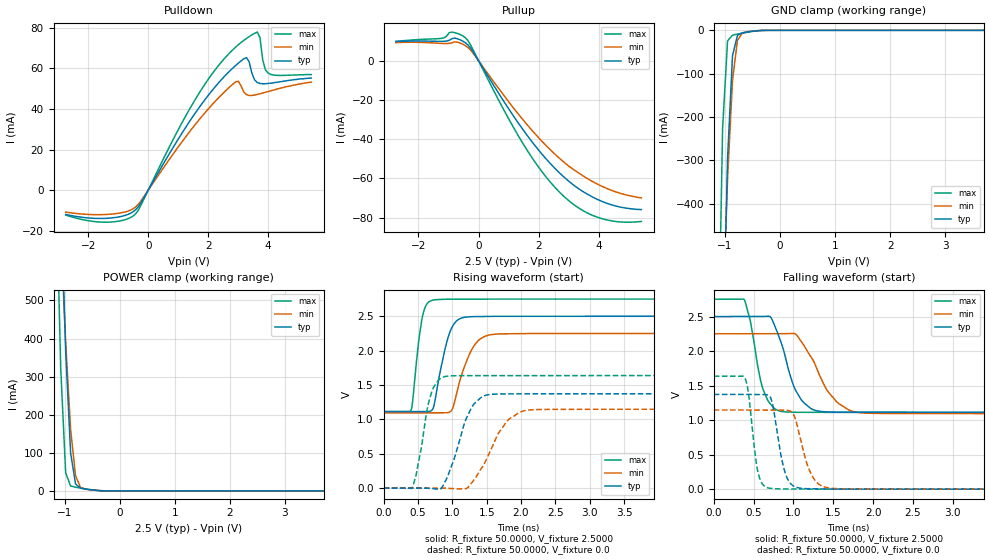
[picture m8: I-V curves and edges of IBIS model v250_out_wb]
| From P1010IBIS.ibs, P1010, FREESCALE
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[Model] v250_out_wb
|   Model v250_out_wb
| This model has derived from v250_wb
| Only applicable curves and parameters are copied
Model_type Output
Polarity   Non-Inverting
Enable   Active-High
Vmeas =  1.2500V
Cref =   0.0F
Rref =   50.0000
Vref =   1.2500V
C_comp   2.1221pF   1.9600pF   2.4667pF
[Temperature Range]   85.0000   0.1250k   -40.0000
[Voltage Range]   2.5000V   2.2500V   2.7500V
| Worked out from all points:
|   slope of the pulldown table from 0 to 0.375 V, typ, clamps not added: 38.9 ohm
|   slope of the pullup table from 0 to 0.375 V, typ, clamps not added: 39.9 ohm
|   GND clamp passes 1 mA (typ) near -0.40 V on its own axis
|   POWER clamp passes 1 mA (typ) near -0.37 V on its own axis
|   rising waveform, R_fixture 50.0000, V_fixture 2.5000: 20-80 % time 180ps typ, 235ps min, 112ps max; typ from 1.11 V to 2.5 V
|   rising waveform, R_fixture 50.0000, V_fixture 0.0: 20-80 % time 275ps typ, 371ps min, 177ps max; typ from 0 V to 1.37 V
|   falling waveform, R_fixture 50.0000, V_fixture 2.5000: 20-80 % time 234ps typ, 336ps min, 160ps max; typ from 2.5 V to 1.11 V
|   falling waveform, R_fixture 50.0000, V_fixture 0.0: 20-80 % time 127ps typ, 169ps min, 96.5ps max; typ from 1.37 V to 0 V
[Pulldown]
|Voltage   I(typ)   I(min)   I(max)
-2.75V    -11.96mA   -10.79mA   -12.27mA
-1.4V     -13.85mA   -11.95mA   -15.75mA
-410mV    -9.504mA   -8.167mA   -11.5mA
1.3V      32.04mA    27.19mA    37.83mA
2.47V     54.84mA    47.31mA    63.54mA
3.01V     62.54mA    53.57mA    71.61mA
3.28V     65.25mA    47.01mA    74.69mA
3.55V     54.3mA     46.83mA    77.2mA
3.73V     52.51mA    47.45mA    75.09mA
3.82V     52.38mA    47.81mA    64.2mA
4V        52.52mA    48.55mA    57.65mA
5.44V     55.2mA     53.18mA    56.9mA
[Pullup]
|Voltage   I(typ)   I(min)   I(max)
-2.75V    9.9mA      9.29mA     9.9mA
-1.25V    9.96mA     8.92mA     11.45mA
-890mV    11.28mA    9.24mA     14.69mA
-440mV    9.214mA    7.771mA    11.81mA
-260mV    6.366mA    5.376mA    7.908mA
1.45V     -34.57mA   -29.59mA   -41.58mA
2.08V     -47.11mA   -40.62mA   -56.03mA
2.62V     -56.14mA   -48.79mA   -65.9mA
3.25V     -64.44mA   -56.41mA   -74.27mA
3.88V     -70.19mA   -62.34mA   -79.38mA
4.6V      -74.22mA   -67.05mA   -82.03mA
5.41V     -75.87mA   -69.91mA   -81.94mA
[GND_clamp]
|Voltage   I(typ)   I(min)   I(max)
-2.75V    -14.95A    -8.916A    -17.97A
-1.13V    -1.387A    -1.039A    -846.5mA
-1.04V    -775.3mA   -667.5mA   -226.6mA
-950mV    -294.9mA   -343.6mA   -24.45mA
-860mV    -58.51mA   -114.8mA   -11.13mA
-770mV    -11.55mA   -23.09mA   -8.664mA
-680mV    -5.737mA   -6.117mA   -6.48mA
-590mV    -3.79mA    -3.141mA   -4.402mA
-230mV    -44.51uA   -32.23uA   -16.96uA
5.44V     0A         0A         0A
[POWER_clamp]
|Voltage   I(typ)   I(min)   I(max)
-2.69V    11.16A     7.25A      12.69A
-1.16V    1.281A     1.002A     850.9mA
-1.07V    788.5mA    681.3mA    324.6mA
-980mV    368.1mA    391mA      47.84mA
-890mV    99.61mA    161.5mA    12.91mA
-800mV    18.31mA    39.69mA    9.783mA
-710mV    7.241mA    9.319mA    7.51mA
-620mV    4.876mA    4.494mA    5.346mA
-260mV    201.3uA    213.5uA    41.93uA
5.5V      0A         0A         0A
[Ramp]
| variable   typ   min   max
dV/dt_r  0.8231/0.2751n   0.6881/0.3712n   0.9819/0.1767n
dV/dt_f  0.8322/0.2342n   0.6935/0.3357n   0.9831/0.1602n
R_load = 50.0000
[Rising Waveform]
R_fixture= 50.0000
V_fixture= 2.5000
V_fixture_min= 2.2500
V_fixture_max= 2.7500
|time   V(typ)   V(min)   V(max)
0s        1.113V     1.094V     1.111V
400.6ps   1.113V     1.094V     1.137V
560.3ps   1.113V     1.094V     2.472V
706.3ps   1.136V     1.094V     2.732V
943.6ps   2.21V      1.1V       2.747V
1.017ns   2.375V     1.193V     2.748V
1.136ns   2.474V     1.651V     2.748V
1.331ns   2.494V     2.091V     2.749V
1.563ns   2.498V     2.232V     2.749V
5ns       2.5V       2.25V      2.75V
[Rising Waveform]
R_fixture= 50.0000
V_fixture= 0.0
V_fixture_min= 0.0
V_fixture_max= 0.0
|time   V(typ)   V(min)   V(max)
0s        11.46uV    23.25uV    1.779uV
414.3ps   -36.43uV   5.787uV    4.619mV
533.5ps   -83.29uV   -7.474uV   499.9mV
655.9ps   -2.986mV   -23.92uV   1.248V
866.1ps   37.64mV    -431.1uV   1.615V
1.261ns   1.138V     51.92mV    1.636V
1.487ns   1.35V      397.7mV    1.636V
1.777ns   1.37V      949.1mV    1.636V
2.038ns   1.371V     1.122V     1.636V
5ns       1.372V     1.147V     1.637V
[Falling Waveform]
R_fixture= 50.0000
V_fixture= 2.5000
V_fixture_min= 2.2500
V_fixture_max= 2.7500
|time   V(typ)   V(min)   V(max)
0s        2.5V       2.25V      2.75V
384.1ps   2.5V       2.25V      2.741V
614.3ps   2.501V     2.25V      1.459V
713.7ps   2.491V     2.25V      1.23V
834.2ps   2.159V     2.25V      1.13V
1.024ns   1.439V     2.248V     1.114V
1.293ns   1.135V     1.742V     1.112V
1.539ns   1.116V     1.269V     1.112V
1.803ns   1.114V     1.112V     1.112V
5ns       1.113V     1.094V     1.111V
[Falling Waveform]
R_fixture= 50.0000
V_fixture= 0.0
V_fixture_min= 0.0
V_fixture_max= 0.0
|time   V(typ)   V(min)   V(max)
0s        1.372V     1.147V     1.637V
390.9ps   1.371V     1.147V     1.611V
550.8ps   1.371V     1.146V     265.7mV
677.1ps   1.363V     1.146V     19.64mV
737.3ps   1.231V     1.146V     9.081mV
895.4ps   237.2mV    1.146V     2.145mV
1.037ns   25.61mV    965.5mV    1.373mV
1.209ns   5.635mV    249.6mV    860uV
1.418ns   1.605mV    22.47mV    496.2uV
5ns       98.66uV    144.2uV    46.47uV
